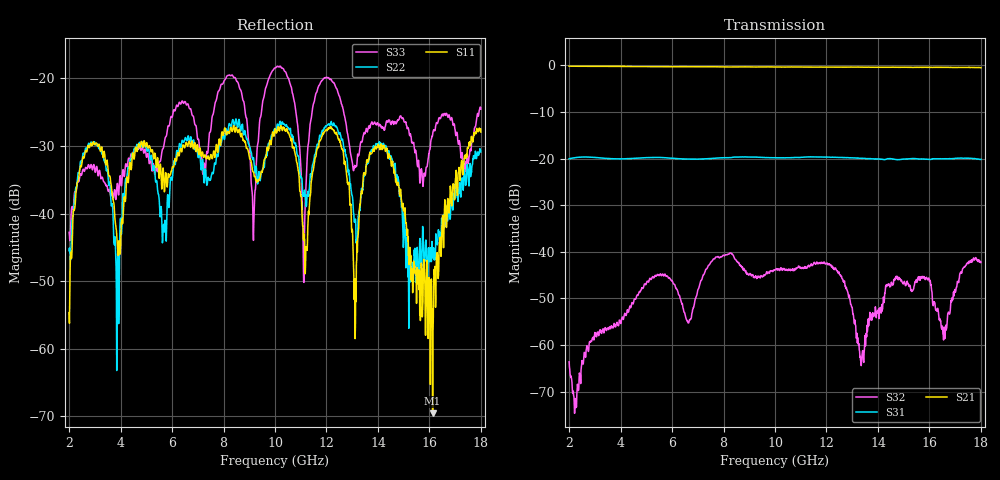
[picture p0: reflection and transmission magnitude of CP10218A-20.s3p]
! Amtery
! Email: info@amtery.com
! Phone: 886-2-2883-7839
! Model Number: CP10218A-20
! 3-port S-parameter measurement data for Directional Coupler
! Frequency Range: 2 GHz to 18 GHz
! Port 1: Input
! Port 2: Output
! Port 3: Coupled
# Hz S db R 50
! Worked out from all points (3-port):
!   1281 points, 2 GHz to 18 GHz, reference 50 ohm
!   strongest paths, dB at 2 GHz, 6 GHz, 10 GHz, 14 GHz, 18 GHz:
!     S21: -0.2, -0.3, -0.3, -0.4, -0.5
!     S31: -20.0, -19.9, -19.8, -20.1, -20.2
!     S32: -63.6, -46.2, -43.9, -53.2, -42.3
!   lowest |S11| = -69.6 dB at 16.12 GHz (marker M1), VSWR 1.00, Z = 50 - j0.0331 ohm
!   |S11| at or under -10 dB: start of sweep to end of sweep
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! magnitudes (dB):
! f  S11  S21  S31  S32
! 2 GHz  -54.7  -0.2  -20.0  -63.6
! 2.788 GHz  -30.2  -0.2  -19.7  -59.3
! 3.875 GHz  -44.5  -0.2  -20.0  -55.6
! 10 GHz  -27.5  -0.3  -19.8  -43.9
! 11.11 GHz  -44.0  -0.4  -19.7  -43.4
! 11.84 GHz  -28.5  -0.4  -19.7  -42.4
! 13.1 GHz  -49.6  -0.4  -19.9  -54.6
! 14.19 GHz  -30.4  -0.4  -20.2  -51.4
! 16.12 GHz  -69.6  -0.4  -20.0  -51.1
! 18 GHz  -27.9  -0.5  -20.2  -42.3
